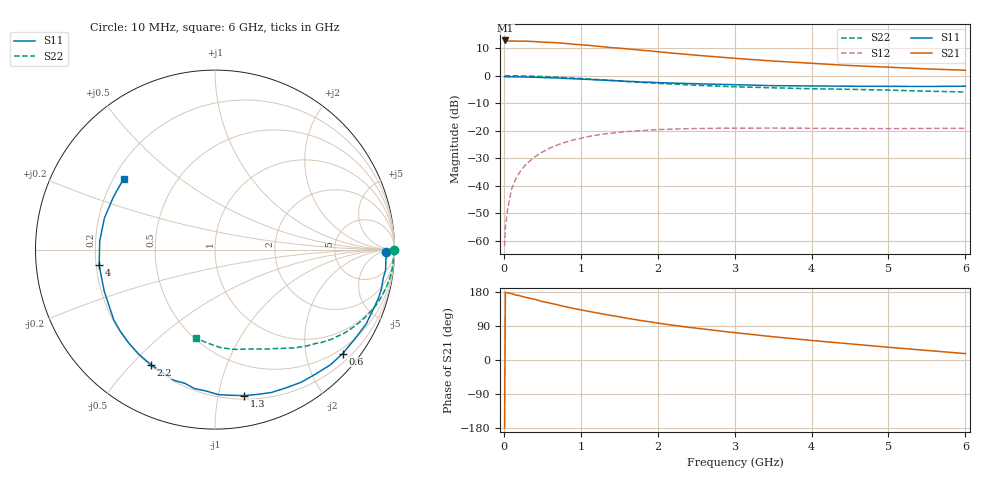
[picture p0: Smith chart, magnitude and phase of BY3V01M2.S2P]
! SIEMENS Small Signal Semiconductors
! BFY420
! Si NPN RF SIEGET Grounded Emitter Transistor in MICRO-X
! VCE = 3 V  IC = 1.2 mA
! Common Emitter S-Parameters:  October  1996
# GHz  S  MA  R  50
!  f  S11  S21  S12  S22
! GHz  MAG  ANG  MAG  ANG  MAG  ANG  MAG  ANG
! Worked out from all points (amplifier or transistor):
!   36 points, 10 MHz to 6 GHz, reference 50 ohm
!   highest |S21| = 12.8 dB at 20 MHz (marker M1)
!   |S21| within 3 dB of that: start of sweep to 1.58 GHz
!   unconditionally stable (mu >= 1): 4.408 GHz to end of sweep
!   at 250 MHz: K = 0.05, MSG = 23.0 dB, |S12| = -33.4 dB
!   at 1.4 GHz: K = 0.21, MSG = 15.6 dB, |S12| = -20.9 dB
!   at 6 GHz: K = 1.32, MAG = 7.2 dB, |S12| = -19.1 dB
!   S11 on the Smith chart (normalised r, x): 10 MHz: 39, -12; 600 MHz: 0.38, -2.76; 1.3 GHz: 0.23, -1.20; 2.2 GHz: 0.20, -0.57; 4 GHz: 0.21, -0.06; 6 GHz: 0.24, +0.32
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0.01  0.9541 -0.8  4.328 -179.5  0.0008 98.4  0.9993 -0.2
0.02  0.9606 -1.5  4.368 178.7  0.0018 84.2  0.9999 -0.6
0.05  0.9537 -3.2  4.262 177.0  0.0038 87.2  0.9981 -1.6
0.1  0.9573 -6.8  4.264 175.3  0.0087 84.7  0.9949 -3.2
0.15  0.9504 -9.8  4.257 171.6  0.0129 83.0  0.9941 -4.7
0.2  0.9529 -13.1  4.241 169.9  0.0171 82.1  0.9936 -6.2
0.3  0.9441 -19.6  4.233 164.5  0.0255 78.4  0.9868 -9.3
0.4  0.9386 -26.1  4.164 160.2  0.0334 73.7  0.9775 -12.3
0.5  0.9248 -32.6  4.068 154.3  0.041 71.0  0.9664 -15.3
0.6  0.9174 -39.2  4.032 150.2  0.0486 67.1  0.9542 -18.2
0.8  0.8917 -51.0  3.855 140.8  0.0618 59.7  0.921 -23.7
1.1  0.856 -68.4  3.568 128.5  0.0786 50.3  0.8711 -31.0
1.3  0.8297 -78.6  3.345 121.0  0.0873 44.5  0.8352 -35.4
1.6  0.7885 -93.9  3.074 110.0  0.0964 36.9  0.7844 -41.4
1.8  0.7638 -102.7  2.892 103.5  0.1009 32.7  0.7548 -44.6
2.2  0.7342 -119.0  2.566 91.7  0.107 25.2  0.7052 -51.0
2.8  0.6964 -139.3  2.181 76.7  0.1111 17.1  0.6437 -58.9
3.5  0.6592 -159.5  1.847 61.4  0.112 10.9  0.6017 -67.1
4  0.6514 -172.3  1.682 51.6  0.1109 7.9  0.5794 -73.1
4.5  0.6441 175.8  1.531 42.6  0.1099 5.6  0.5656 -79.4
5.5  0.6374 152.8  1.328 25.2  0.1101 4.9  0.5235 -94.1
6  0.6444 142.2  1.256 16.9  0.1109 5.5  0.5062 -102.3
